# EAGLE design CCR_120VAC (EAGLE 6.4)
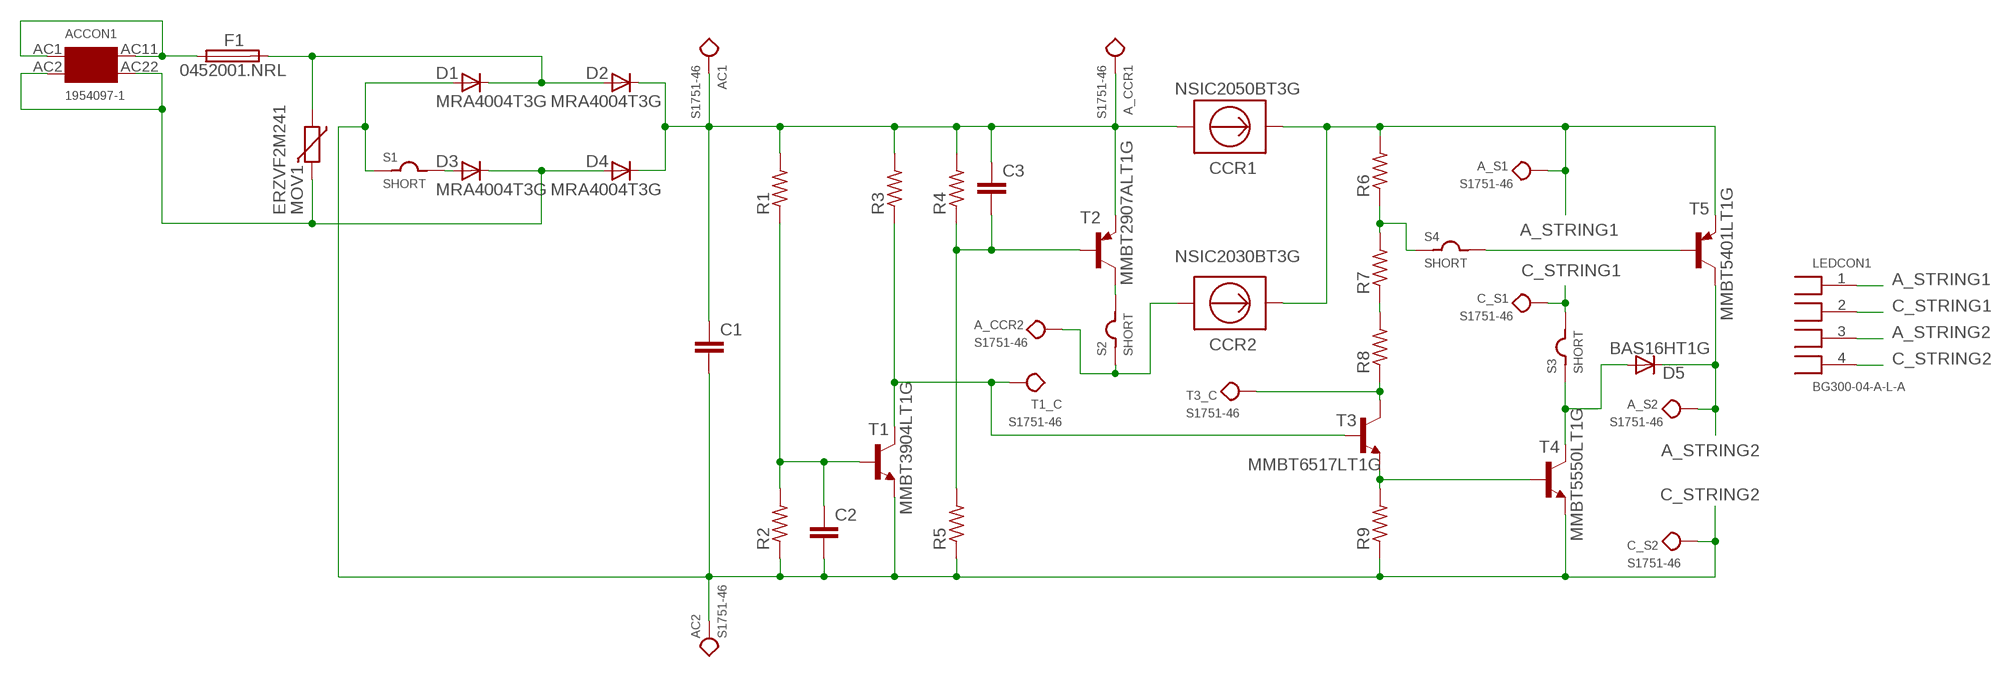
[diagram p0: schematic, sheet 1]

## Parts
A_CCR1  S1751-46  [TEST_SMT]
A_CCR2  S1751-46  [TEST_SMT]
A_S1  S1751-46  [TEST_SMT]
A_S2  S1751-46  [TEST_SMT]
AC1  S1751-46  [TEST_SMT]
AC2  S1751-46  [TEST_SMT]
ACCON1  1954097-1  [LEDCON_SMT]
C1  C-EUC1206K  [C1206K]
C2  C-EUC0805K  [C0805K]
C3  C-EUC0805K  [C0805K]
C_S1  S1751-46  [TEST_SMT]
C_S2  S1751-46  [TEST_SMT]
CCR1  NSIC2050BT3G  [SMB]
CCR2  NSIC2030BT3G  [SMB]
D1  MRA4004T3G  [SMA]
D2  MRA4004T3G  [SMA]
D3  MRA4004T3G  [SMA]
D4  MRA4004T3G  [SMA]
D5  BAS16HT1G  [SOD323-R]
F1  0452001.NRL  [SMTFUSE]
LEDCON1  BG300-04-A-L-A  [LEDCON_4_F]
MOV1  ERZVF2M241  [CU3225K]
R1  R-US_R1206  [R1206]
R2  R-US_R1206  [R1206]
R3  R-US_R1206  [R1206]
R4  R-US_R1206  [R1206]
R5  R-US_R1206  [R1206]
R6  R-US_R1206  [R1206]
R7  R-US_R1206  [R1206]
R8  R-US_R1206  [R1206]
R9  R-US_R1206  [R1206]
S1  SHORT  [R2010]
S2  SHORT  [R2010]
S3  SHORT  [R2010]
S4  SHORT  [R2010]
T1  MMBT3904LT1G  [SOT23]
T1_C  S1751-46  [TEST_SMT]
T2  MMBT2907ALT1G  [SOT23]
T3  MMBT6517LT1G  [SOT23]
T3_C  S1751-46  [TEST_SMT]
T4  MMBT5550LT1G  [SOT23]
T5  MMBT5401LT1G  [SOT23]

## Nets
A_STRING1: A_S1.P$1 CCR1.C CCR2.C LEDCON1.1 R6.2 T5.2(E)
A_STRING2: A_S2.P$1 D5.C LEDCON1.3 T5.3(C)
C_STRING1: C_S1.P$1 LEDCON1.2 S3.2
C_STRING2: AC2.P$1 C1.2 C2.2 C_S2.P$1 D1.A LEDCON1.4 R2.1 R5.1 R9.1 S1.1 T1.2(E) T4.2(E)
N$1: ACCON1.AC1 ACCON1.AC11 F1.P$1
N$2: ACCON1.AC2 ACCON1.AC22 D3.C D4.A MOV1.2
N$3: D1.C D2.A F1.P$2 MOV1.1
N$4: R6.1 R7.2 S4.1
N$5: C2.1 R1.1 R2.2 T1.1(B)
N$6: D3.A S1.2
N$7: A_CCR1.P$1 AC1.P$1 C1.1 C3.1 CCR1.A D2.C D4.C R1.2 R3.2 R4.2 T2.2(E)
N$8: R3.1 T1.3(C) T1_C.P$1 T3.1(B)
N$9: C3.2 R4.1 R5.2 T2.1(B)
N$10: R7.1 R8.2
N$11: R8.1 T3.3(C) T3_C.P$1
N$12: A_CCR2.P$1 CCR2.A S2.1
N$13: S2.2 T2.3(C)
N$14: R9.2 T3.2(E) T4.1(B)
N$15: D5.A S3.1 T4.3(C)
N$16: S4.2 T5.1(B)

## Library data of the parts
A_CCR1 A_CCR2 A_S1 A_S2 AC1 AC2 C_S1 C_S2 T1_C T3_C = CCR_120VAC_LIB:S1751-46
ACCON1 = CCR_120VAC_LIB:1954097-1
C1-C3 = resistor:C-EU: CAPACITOR, European symbol
CCR1 = CCR_120VAC_LIB:NSIC2050BT3G
CCR2 = CCR_120VAC_LIB:NSIC2030BT3G
D1-D4 = CCR_120VAC_LIB:MRA4004T3G
D5 = CCR_120VAC_LIB:BAS16HT1G
F1 = CCR_120VAC_LIB:0452001.NRL
LEDCON1 = CCR_120VAC_LIB:BG300-04-A-L-A
MOV1 = CCR_120VAC_LIB:ERZVF2M241
R1-R9 = resistor:R-US_: RESISTOR, American symbol
S1-S4 = CCR_120VAC_LIB:SHORT
T1 = CCR_120VAC_LIB:MMBT3904LT1G
T2 = CCR_120VAC_LIB:MMBT2907ALT1G
T3 = CCR_120VAC_LIB:MMBT6517LT1G
T4 = CCR_120VAC_LIB:MMBT5550LT1G
T5 = CCR_120VAC_LIB:MMBT5401LT1G

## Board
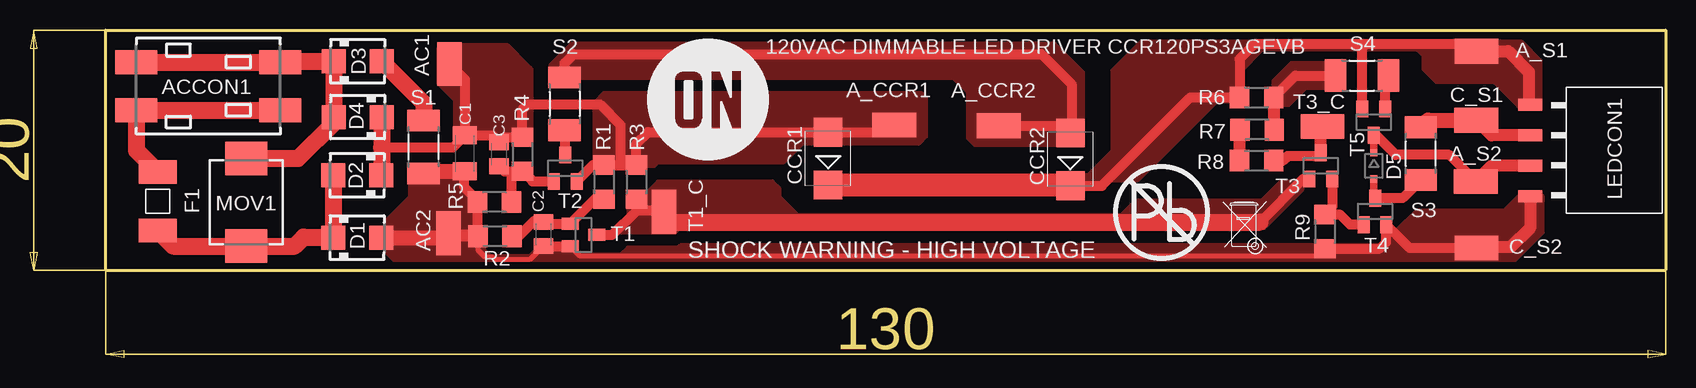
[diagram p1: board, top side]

Size 136.3 x 27.3 mm. Coordinates in mm from the lower left corner, seen from the top.
Outline: 6.3,7.3 6.3,27.3 136.3,27.3 136.3,7.3 6.3,7.3
Copper layers (1*16): Top 0.035mm / dielectric 1.5mm / Bottom 0.035mm
Design rules "default": minimum track width 10mil, minimum drill 24mil, track to track 8mil, track to pad 8mil, pad to pad 8mil, via to via 8mil, smd to smd 8mil, copper to edge 1mil, drill to drill 8mil, minimum pad ring 10mil, minimum via ring 8mil, stop-mask expansion 4mil, vias tented up to drill 0mil, thermal gap 10mil

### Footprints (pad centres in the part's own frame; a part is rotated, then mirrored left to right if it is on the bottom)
TEST_SMT = smd 3.65 x 2.05: P$1 0,0
LEDCON_SMT = smd 3.5 x 2: AC1 -6,2; AC2 -6,-2; AC11 6,2; AC22 6,-2
C1206K = smd 1.5 x 2: 1 -1.5,0; 2 1.5,0
C0805K = smd 1.3 x 1.6: 1 -1,0; 2 1,0
SMB = smd 2.4 x 2.4: A 2.2,0; C -2.2,0
SMA = smd 2 x 2: A 2,0; C -2,0
SOD323-R = smd 0.6 x 0.6: A 1.1,0; C -1.1,0
SMTFUSE = smd 1.96 x 3.15: P$1 -2.45,0; P$2 2.45,0
LEDCON_4_F = smd 2 x 1: 1 0,2.54; 2 0,0; 3 0,-2.54; 4 0,-5.08
CU3225K = smd 2.8 x 3.5: 1 -3.65,0; 2 3.65,0
R1206 = smd 1.6 x 1.803: 1 -1.422,0; 2 1.422,0
R2010 = smd 1.8 x 2.7: 1 -2.2,0; 2 2.2,0
SOT23 = smd 1 x 1.4: 1 -0.95,-1.1; 2 0.95,-1.1; 3 0,1.1

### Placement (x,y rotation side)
A_CCR1  72.01,19.38 0 top
A_CCR2  80.73,19.32 180 top
A_S1  120.54,25.53 0 top
A_S2  120.49,14.68 0 top
AC1  34.97,24.46 90 top
AC2  34.89,10.36 90 top
ACCON1  14.86,22.62 180 top
C1  36.24,17.01 270 top
C2  42.79,10.29 270 top
C3  39.09,16.95 270 top
C_S1  120.52,19.78 0 top
C_S2  120.54,9.13 0 top
CCR1  66.5,16.59 90 top
CCR2  86.7,16.52 90 top
D1  27.25,10 0 top
D2  27.27,15.2 180 top
D3  27.31,24.7 0 top
D4  27.31,20.05 180 top
D5  111.99,15.98 270 top
F1  10.65,13.03 270 top
LEDCON1  125,18.52 0 top
MOV1  18.02,12.95 90 top
R1  47.84,14.63 90 top
R2  38.75,10.11 0 top
R3  50.54,14.62 90 top
R4  41.04,16.94 90 top
R5  38.71,12.96 0 top
R6  102.22,21.69 180 top
R7  102.26,18.99 0 top
R8  102.22,16.41 180 top
R9  107.91,10.5 90 top
S1  32.8,17.55 90 top
S2  44.55,21.15 270 top
S3  115.9,17 90 top
S4  111,23.5 0 top
T1  46.13,10.22 270 top
T1_C  52.83,12.16 270 top
T2  44.6,15.78 0 top
T3  107.57,15.98 0 top
T3_C  107.71,19.27 180 top
T4  112.09,12.18 0 top
T5  111.99,19.62 180 top
U$1  [ON2]  56.5,21.5 0 top
U$2  [PB1]  94.3,12.1 0 top
U$3  [BIN2]  101.2,10.9 0 top

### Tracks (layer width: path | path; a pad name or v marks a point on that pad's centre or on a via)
A_STRING1
  Top 0.813: 86.63,14.39 CCR2.C 89.32,14.32 96.69,21.69 R6.2 100.8,24.9 102,26.1 111.3,26.1 | A_S1.P$1 119.97,26.1 111.3,26.1 | T5.2 111.04,25.84 111.3,26.1
  Top 1.016: A_S1.P$1 123.17,25.53 124.9,23.8 124.9,21.16 LEDCON1.1
  Top 1.93: CCR1.C 86.63,14.39
  pour Top (no thermals): 87.5,15.3 88.2,15.3 90.2,17.3 90.2,24 92.4,26.2 92.5,26.3 92.6,26.4 124.3,26.4 125.9,24.8 125.9,20.8 125.8,20.7 124.2,20.7 124,20.9 122,22.9 117.2,22.9 116.1,24 116.1,25.1 115.6,25.6 102.7,25.6 100.9,23.8 100.9,21.3 98.9,21.3 96.5,18.9 92.3,14.7 91.5,14.7 89.7,14.7 89,14 87.7,14 87.5,14.2
A_STRING2
  Top 0.61: D5.C T5.3
  Top 0.813: A_S2.P$1 118.27,16.9 113.8,16.9 112.18,18.52 T5.3
  Top 1.016: LEDCON1.3 121.79,15.98 A_S2.P$1
C_STRING1
  Top 1.016: LEDCON1.2 121.78,18.52 C_S1.P$1
  Top 1.27: S3.2 116.48,19.78 C_S1.P$1
C_STRING2
  Top 0.406: T1.2 45.8,8.5 107.33,8.5 R9.1 | R2.1 37.33,8.97 37.9,8.4 38.5,8.4 38.7,8.2 41.7,8.2 C2.2
  Top 0.813: R2.1 37.29,10.15 R5.1 37.29,13.11 36.2,14.2 36.2,15.47 C1.2 | C2.2 45.01,9.29 T1.2 | R9.1 112.48,9.08 113,9.6 113,11.04 T4.2 114.99,9.13 C_S2.P$1
  Top 1.016: 37.29,10.15 35.1,10.15 AC2.P$1 | LEDCON1.4 125,10.8 123.4,9.2 120.61,9.2 C_S2.P$1
  Top 1.27: S1.1 32.96,15.51 C1.2 | D1.A 34.53,10 AC2.P$1
  pour Top (no thermals): 31.6,15.7 31.6,13.4 29.6,11.4 29.6,8.8 30.2,8.2 30.3,8.1 123.8,8.1 126.1,10.4 126.1,13.5 125.8,13.8 124.3,13.8 122.8,12.3 115.5,12.3 113.8,10.6 113.8,10.5 112.7,9.4 54.2,9.4 54,9.2 49.8,9.2 49.2,8.6 45.8,8.6 45,9.4 42.5,9.4 41.6,8.5 38.4,8.5 37.9,9 37.9,10.1 37.4,10.6 37.4,13.3 35.6,15.1 35.6,15.4 35.2,15.8 31.7,15.8
N$1
  Top 1.422: ACCON1.AC1 ACCON1.AC11 8.86,17.27 F1.P$1
N$2
  Top 1.422: ACCON1.AC22 ACCON1.AC2 20.94,24.7 D3.C D4.A 25.3,19.55 22.35,16.6 MOV1.2
N$3
  Top 1.422: D2.A 25.27,10.02 D1.C 25.2,10.05 22.8,10.05 22.05,9.3 MOV1.1 11.93,9.3 F1.P$2
N$4
  Top 0.813: R6.1 105.45,23.5 S4.1
  Top 1.016: R7.2 103.68,21.65 R6.1
  pour Top (no thermals): 103.6,22.5 103.6,23.1 105.1,24.6 109.4,24.6 109.4,22.4 106.3,22.4 104.9,21 103.6,21
N$5
  Top 0.813: R1.1 47.07,13.21 T1.1 42.91,11.17 C2.1 42.68,11.4 42,11.4 40.71,10.11 R2.2
N$6
  Top 1.422: D3.A 32.8,21.21 S1.2
N$7
  Top 0.813: C1.1 35.23,17.5 29.31,17.5 | AC1.P$1 36.24,23.19 C1.1 | C1.1 38.53,18.51 C3.1 39.5,18.36 R4.2 41.04,20.64 41.5,21.1 47.5,21.1 49.2,19.4 49.2,16.14 49.3,16.04 | T2.2 46.92,16.05 R1.2 49.3,16.04 | 49.3,16.04 R3.2 50.54,17.84 51.5,18.8 CCR1.A 71.42,18.79 A_CCR1.P$1
  Top 1.422: D4.C 29.31,17.5 29.31,15.24 D2.C
  pour Top (no thermals): 47,16 47,21.3 47.8,22.1 74.3,22.1 74.7,21.7 74.7,18.4 74.1,17.8 64.4,17.8 62.8,16.2 52.3,16.2 52,15.9 47.1,15.9
  pour Top (no thermals): 34.3,26.1 39.8,26.1 41.6,24.3 41.7,24.2 41.8,24.1 41.8,19 41.1,18.3 36.1,18.3 35.4,19 35.4,21.4 34,22.8 34,25.8
N$8
  Top 0.813: T1.3 48.52,10.22 50.6,12.3 | 50.6,12.3 50.6,13.14 R3.1 | 50.6,12.3 52.69,12.3 T1_C.P$1 53.69,11.3 | 102.5,11.3 106.08,14.88 T3.1
  Top 1.422: 53.69,11.3 102.5,11.3
  pour Top (no thermals): 49.2,10.4 53.8,10.4 54.2,10.8 102.9,10.8 106.1,14 106.1,14.5 105.9,14.7 104.2,14.7 102.6,13.1 92.1,13.1 90.9,11.9 64,11.9 62.5,13.4 62.5,14.1 61.9,14.7 52.3,14.7 51.3,13.7 50.7,13.7 49.8,12.8 49.8,11.6 49.2,11
N$9
  Top 0.813: C3.2 39.52,15.52 40.1,15.52 | 40.1,15.52 R4.1 41.88,14.68 T2.1 | R5.2 40.13,15.49 40.1,15.52
N$10
  Top 1.016: R8.2 100.8,18.95 R7.1
N$11
  Top 0.813: T3.3 107.29,16.8 104.8,16.8 104.41,16.41 R8.1
  Top 1.016: T3.3 107.57,19.13 T3_C.P$1
N$12
  Top 0.813: S2.1 44.55,24.55 45.3,25.3 84.3,25.3 86.8,22.8 86.8,18.82 CCR2.A 86.1,19.32 A_CCR2.P$1
  pour Top (no thermals): 44.4,23.3 76.9,23.3 78.1,22.1 78.1,18.3 78.7,17.7 87.6,17.7 87.8,17.9 87.8,23.8 85.4,26.2 45.1,26.2 43.3,24.4 43.3,23.7 43.7,23.3
N$13
  Top 0.813: T2.3 44.6,18.9 S2.2
N$14
  Top 0.813: T4.1 110.02,11.08 109.2,11.9 107.93,11.9 R9.2 108.52,12.53 T3.2
N$15
  Top 0.61: D5.A 111.99,13.38 T4.3
  Top 0.813: S3.1 114.38,13.28 T4.3
N$16
  Top 0.813: T5.1 112.94,23.24 S4.2

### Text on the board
tNames: 120VAC DIMMABLE LED DRIVER CCR120PS3AGEVB | SHOCK WARNING - HIGH VOLTAGE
